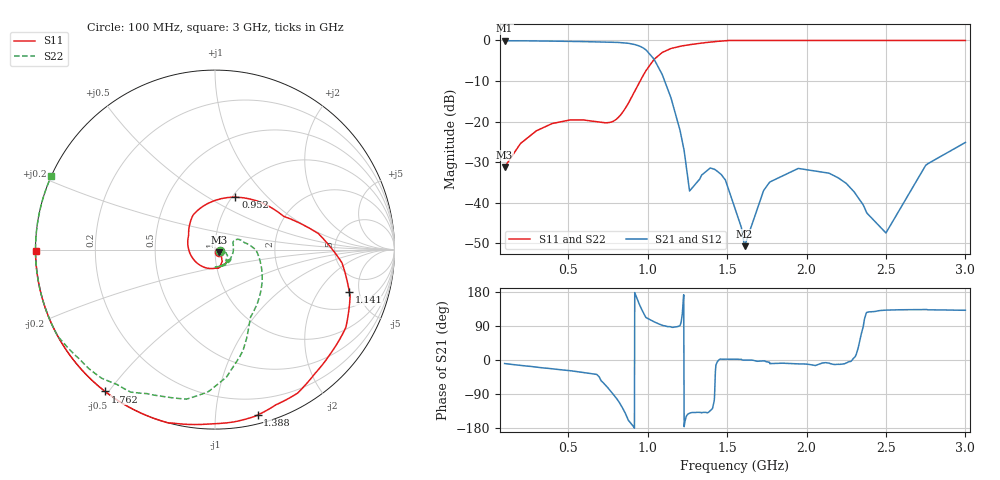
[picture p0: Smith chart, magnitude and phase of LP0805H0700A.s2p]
! AVX THIN FILM OPERATION
! LP0805 High Performance Low Pass Filter P/N  LP0805H0700ASTR
! 28 June 2017
# MHz S dB R 50
!  Frq	S11(dB)	S11(deg)	S21(dB)	S21(deg)	S12(dB)	S12(deg)	S22(dB)	S22(deg)
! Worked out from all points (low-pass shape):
!   501 points, 100 MHz to 3 GHz, reference 50 ohm
!   highest |S21| = -0.07 dB at 100 MHz (marker M1); lowest = -50.8 dB at 1.61 GHz (marker M2)
!   |S21| within 3 dB of the highest: start of sweep to 1.006 GHz
!   lowest |S11| = -31.2 dB at 100 MHz (marker M3), VSWR 1.06, Z = 52.3 - j1.59 ohm
!   |S11| at or under -10 dB: start of sweep to 953.1 MHz
!   |S22| runs from -31.2 to 0.0 dB; largest |S21 - S12| = 0.051
!   S11 on the Smith chart (normalised r, x): 100 MHz: 1.05, -0.03; 952 MHz: 1.04, +0.67; 1.141 GHz: 3.19, -3.98; 1.388 GHz: 0.07, -1.29; 1.762 GHz: 0.00, -0.49; 3 GHz: -0.00, -0.00
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100  -31.24 -33.6  -0.07 -9.4  -0.07 -9.5  -31.24 -16.9
310  -22.11 -59.8  -0.13 -19.4  -0.13 -19.3  -22.11 -29.1
585.8  -19.61 -84.3  -0.27 -32.5  -0.27 -32.7  -19.61 -40.4
694  -20.14 -86.0  -0.36 -43.3  -0.36 -43.5  -20.14 -67.7
811.2222  -19.17 -107.8  -0.48 -105.4  -0.48 -105.6  -19.17 23.7
879  -15.49 150.8  -0.70 -159.2  -0.70 -157.8  -15.49 13.4
915  -12.86 122.6  -0.96 -177.8  -0.96 -174.7  -12.86 -0.5
952  -10.08 68.8  -1.43 143.3  -1.43 144.3  -10.08 -32.9
987.8889  -7.58 28.0  -2.28 113.4  -2.28 114.8  -7.58 -60.7
1068.889  -3.73 0.5  -6.71 95.4  -6.71 94.5  -3.73 -80.4
1140.889  -2.09 -17.6  -13.51 88.1  -13.51 85.7  -2.09 -92.1
1204  -1.43 -30.8  -22.17 90.8  -22.17 89.4  -1.43 -100.8
1264  -1.04 -51.1  -37.15 -140.2  -37.15 -143.1  -1.04 -115.2
1388  -0.43 -75.5  -31.66 -136.2  -31.66 -141.5  -0.43 -130.8
1484.222  -0.06 -102.5  -34.17 2.2  -34.17 -3.8  -0.06 -148.8
1556.667  0.00 -108.0  -42.24 2.0  -42.24 -1.0  0.00 -152.6
1610  0.00 -115.7  -50.76 -0.3  -50.76 -2.9  0.00 -157.6
1762.444  0.00 -127.8  -35.26 -6.0  -35.26 -13.0  0.00 -166.2
2034.222  0.00 -139.1  -32.10 -13.0  -32.10 -11.7  0.00 -174.3
2527.778  0.00 -168.2  -45.65 132.0  -45.65 135.2  0.00 164.3
2765  0.00 -175.7  -30.38 132.4  -30.38 128.8  0.00 158.5
3000  0.00 -179.4  -25.17 131.2  -25.17 125.4  0.00 155.8
